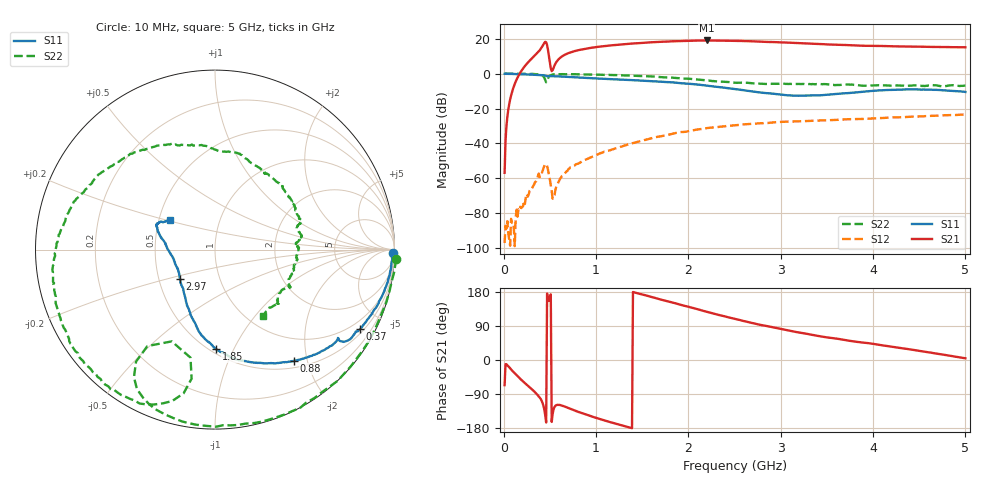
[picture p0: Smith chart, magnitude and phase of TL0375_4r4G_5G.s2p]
! Created Fri Jul 02 06:40:39 2021
# hz S ri R 50
! 2 Port Network Data from SP1.SP block
! freq  reS11  imS11  reS21  imS21  reS12  imS12  reS22  imS22
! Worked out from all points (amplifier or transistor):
!   500 points, 10 MHz to 5 GHz, reference 50 ohm
!   highest |S21| = 19.0 dB at 2.2 GHz (marker M1)
!   |S21| within 3 dB of that: 1.131 GHz to 3.882 GHz (2.75 GHz wide, 110 % of centre)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
!   unconditionally stable (mu >= 1): 35.59 MHz to 136.2 MHz; 142.5 MHz to 188.4 MHz; 194 MHz to end of sweep
!   at 840 MHz: K = 1.71, MAG = 27.3 dB, |S12| = -50.5 dB
!   at 2.51 GHz: K = 1.30, MAG = 20.9 dB, |S12| = -29.6 dB
!   at 5 GHz: K = 1.06, MAG = 17.7 dB, |S12| = -23.3 dB
!   S11 on the Smith chart (normalised r, x): 10 MHz: 46, -83; 370 MHz: 0.64, -3.81; 880 MHz: 0.60, -1.77; 1.85 GHz: 0.53, -0.86; 2.97 GHz: 0.64, -0.23; 5 GHz: 0.57, +0.20
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1e7  0.9896 -0.0183  0.00058 -0.00132  -1.02e-05 -9.64e-06  1.009 -0.0546
1e8  0.973 -0.1404  0.3122 -0.1817  -5.1e-05 1.7e-05  0.8215 -0.5643
2.6e8  0.8894 -0.3319  0.7875 -1.895  -0.0003 7.94e-06  0.1679 -0.9698
3.7e8  0.8091 -0.4428  -0.2215 -4.117  -0.00115 -1.95e-05  -0.2597 -0.9266
4.1e8  0.7742 -0.4735  -1.623 -5.342  -0.00131 0.000254  -0.4001 -0.826
4.3e8  0.7548 -0.4979  -3.475 -5.924  -0.00182 0.000619  -0.4516 -0.7111
4.6e8  0.6952 -0.509  -7.656 -2.046  -0.0011 0.00231  -0.241 -0.5113
4.9e8  0.6872 -0.4934  -2.89 1.303  0.000374 0.00117  -0.1754 -0.8012
5.1e8  0.6814 -0.5026  -1.411 0.1682  0.000168 0.000607  -0.2907 -0.8566
5.4e8  0.667 -0.5197  -0.9484 -1.116  -0.00022 0.000219  -0.4198 -0.8575
6.5e8  0.5894 -0.5685  -1.773 -2.842  -0.00129 -2.67e-05  -0.6373 -0.7208
8.5e8  0.4572 -0.6158  -3.825 -3.173  -0.00308 0.000366  -0.8191 -0.4827
8.8e8  0.4392 -0.6201  -4.095 -3.11  -0.00334 0.000512  -0.8346 -0.4464
1.29e9  0.2324 -0.6299  -6.887 -0.8374  -0.00774 0.00318  -0.8904 -0.0339
1.68e9  0.0701 -0.5896  -7.717 2.66  -0.0123 0.00996  -0.7404 0.3134
1.85e9  0.00737 -0.5553  -7.41 4.213  -0.0135 0.014  -0.6234 0.4352
2.2e9  -0.0965 -0.4439  -5.409 7.127  -0.0123 0.0247  -0.2621 0.5862
2.51e9  -0.1469 -0.3287  -2.722 8.269  -0.00693 0.0324  0.0338 0.5476
2.97e9  -0.1958 -0.165  0.9069 7.91  0.00474 0.0408  0.3459 0.3768
3.34e9  -0.2279 -0.0609  2.921 6.658  0.0149 0.0423  0.4536 0.2188
4.17e9  -0.3215 0.1133  4.949 3.622  0.0363 0.0411  0.4538 -0.0321
5e9  -0.2516 0.1623  5.687 0.4449  0.0618 0.0286  0.2696 -0.3688
